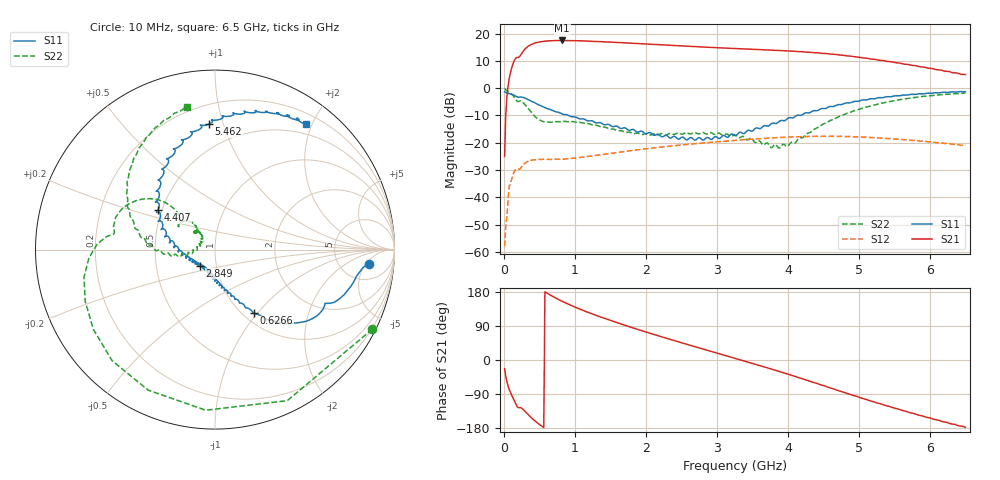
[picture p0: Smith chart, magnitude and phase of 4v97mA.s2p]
!Agilent Technologies,N5230A,MY45000233,A.04.83
!Agilent N5230A: A.04.83
!Date: Friday, August 18, 2006 03:09:01
!Correction: S11(Full 2 Port SOLT,1,2) S21(Full 2 Port SOLT,1,2) S12(Full 2 Port SOLT,1,2) S22(Full 2 Port SOLT,1,2)
!S2P File: Measurements: S11, S21, S12, S22:
# Hz S  dB  R 50
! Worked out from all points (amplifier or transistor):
!   401 points, 10 MHz to 6.5 GHz, reference 50 ohm
!   highest |S21| = 17.5 dB at 821.2 MHz (marker M1)
!   |S21| within 3 dB of that: 302 MHz to 3.297 GHz (2.995 GHz wide, 166 % of centre)
!   unconditionally stable (mu >= 1): start of sweep to end of sweep
!   at 1.081 GHz: K = 1.28, MAG = 18.2 dB, |S12| = -25.3 dB
!   at 3.255 GHz: K = 1.10, MAG = 14.9 dB, |S12| = -19.1 dB
!   at 6.5 GHz: K = 1.06, MAG = 11.5 dB, |S12| = -20.9 dB
!   S11 on the Smith chart (normalised r, x): 10 MHz: 9, -6; 626.5 MHz: 1.12, -0.96; 2.849 GHz: 0.83, -0.15; 4.407 GHz: 0.48, +0.25; 5.462 GHz: 0.33, +0.90; 6.5 GHz: 0.35, +1.90
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1e7  -1.31 -5.5  -25.01 -23.2  -57.86 -170.3  -0.15 -26.8
7.49e7  -2.01 -13.0  3.48 -77.7  -35.70 137.4  -1.48 -132.8
1.398e8  -2.54 -21.5  9.70 -104.9  -30.83 86.7  -3.04 -176.1
3.0205e8  -3.71 -37.4  14.46 -136.3  -27.35 49.5  -6.17 145.0
4.48075e8  -5.55 -49.6  16.58 -162.4  -26.19 28.9  -10.61 135.4
6.2655e8  -7.62 -58.5  17.31 174.2  -26.09 16.2  -12.42 146.4
8.2125e8  -9.44 -63.1  17.45 154.8  -25.96 10.5  -12.22 146.5
1.097075e9  -11.25 -71.2  17.31 132.2  -25.31 5.5  -12.63 137.4
1.324225e9  -12.70 -77.2  17.07 116.0  -24.55 1.0  -13.74 131.3
1.5676e9  -13.93 -83.8  16.76 100.1  -23.66 -5.0  -15.26 128.9
1.875875e9  -16.10 -90.2  16.35 81.3  -22.59 -13.7  -16.45 134.3
2.18415e9  -16.99 -100.0  15.90 63.3  -21.71 -23.8  -17.09 138.6
2.849375e9  -18.18 -133.9  14.99 26.5  -19.98 -47.6  -16.81 136.2
3.255e9  -17.40 -151.6  14.50 4.6  -19.12 -63.4  -17.19 132.4
3.74175e9  -13.62 176.0  13.95 -22.5  -18.26 -84.1  -21.19 144.3
4.342075e9  -8.47 146.1  13.04 -58.1  -17.69 -112.3  -15.75 -167.6
4.406975e9  -8.26 145.1  12.94 -61.8  -17.62 -115.2  -14.57 -172.5
4.8775e9  -5.36 120.1  11.73 -90.7  -17.71 -138.9  -8.86 175.9
5.42915e9  -3.15 96.0  9.72 -122.5  -18.46 -164.8  -4.93 149.4
5.4616e9  -3.10 92.6  9.63 -124.8  -18.44 -166.7  -4.80 148.8
5.932125e9  -1.99 73.8  7.61 -150.1  -19.44 172.5  -2.99 126.2
6.5e9  -1.29 54.2  4.94 -177.6  -20.95 149.3  -1.85 101.2
